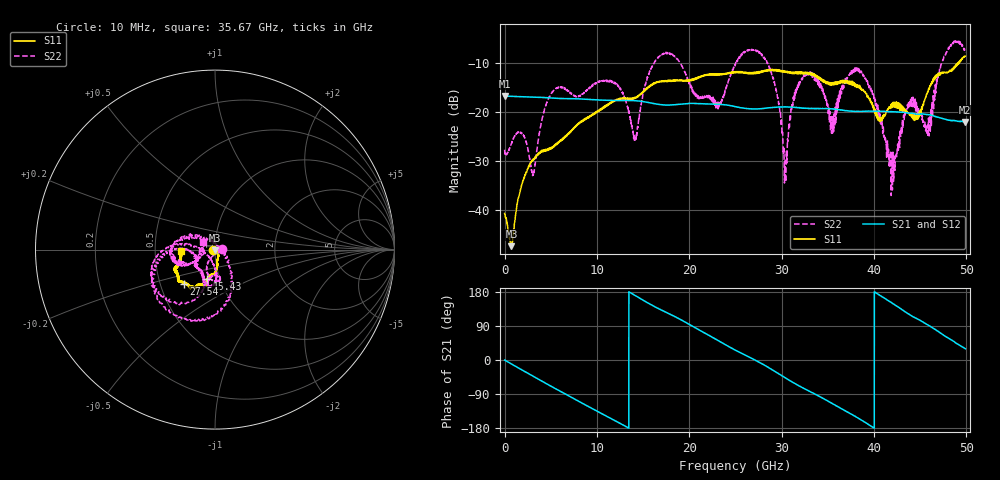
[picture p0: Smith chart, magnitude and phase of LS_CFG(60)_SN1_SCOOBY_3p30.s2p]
!Keysight Technologies,N5245B,MY58422026,A.13.80.08
!Date: Thursday, March 19, 2020 23:45:45
!Correction: S11(Full 2 Port(1,2))
!S21(Full 2 Port(1,2))
!S12(Full 2 Port(1,2))
!S22(Full 2 Port(1,2))
!S2P File: Measurements: S11, S21, S12, S22:
# Hz S DB R 50.0
!freq dBS11 angS11 dBS21 angS21 dBS12 angS12 dBS22 angS22
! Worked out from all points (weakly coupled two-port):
!   4991 points, 10 MHz to 49.91 GHz, reference 50 ohm
!   highest |S21| = -16.79 dB at 10 MHz (marker M1); lowest = -22.1 dB at 49.82 GHz (marker M2)
!   lowest |S11| = -47.4 dB at 750 MHz (marker M3), VSWR 1.01, Z = 49.8 - j0.367 ohm
!   |S11| at or under -10 dB: start of sweep to 49.13 GHz; 49.16379 GHz to 49.2268 GHz (63.01 MHz wide, 0.128 % of centre)
!   |S22| runs from -37.0 to -5.5 dB; largest |S21 - S12| = 0.0015
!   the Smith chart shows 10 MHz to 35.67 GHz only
!   S11 on the Smith chart (normalised r, x): 10 MHz: 0.98, -0.01; 15.43 GHz: 0.87, -0.30; 27.54 GHz: 0.66, -0.27; 35.67 GHz: 0.68, -0.01
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1e7  -40.71 -162.0  -16.79 -0.3  -16.77 -0.3  -27.72 0.9
7.5e8  -47.36 -120.7  -16.84 -10.5  -16.83 -10.5  -26.45 -29.2
2.8e9  -30.48 -55.0  -16.97 -38.6  -16.96 -38.6  -30.48 -29.9
5.15e9  -27.22 -66.6  -17.19 -70.8  -17.19 -70.7  -16.01 -101.9
8.33e9  -22.10 -81.1  -17.39 -113.0  -17.39 -112.9  -16.54 -95.8
1.208e10  -17.60 -89.0  -17.69 -161.5  -17.68 -161.4  -14.21 -91.3
1.412e10  -17.23 -97.6  -17.73 170.7  -17.73 170.8  -25.78 -138.5
1.543e10  -15.37 -104.3  -18.05 151.8  -18.05 151.9  -13.32 171.2
1.665e10  -13.95 -104.2  -18.46 135.9  -18.46 135.9  -8.93 -165.7
2.312e10  -12.50 -118.4  -18.44 51.7  -18.44 51.9  -19.39 -155.5
2.496e10  -12.00 -123.7  -18.91 26.5  -18.90 26.7  -10.55 -171.5
2.754e10  -11.83 -132.3  -19.38 -5.4  -19.38 -5.2  -7.82 -103.8
2.931e10  -11.51 -140.8  -19.07 -30.6  -19.07 -30.4  -14.71 -60.8
3.039e10  -11.81 -144.1  -19.01 -46.9  -19.01 -46.7  -31.25 44.2
3.148e10  -11.96 -150.0  -19.08 -62.6  -19.08 -62.3  -15.91 147.5
3.328e10  -12.31 -156.6  -19.31 -85.9  -19.32 -85.5  -12.25 -166.8
3.567e10  -14.38 -177.5  -19.43 -117.1  -19.37 -116.7  -22.23 147.2
3.839e10  -15.07 174.3  -19.93 -154.6  -19.87 -154.9  -11.33 -162.4
4.16e10  -19.12 106.2  -19.95 156.1  -19.97 156.0  -28.20 83.5
4.675e10  -12.50 7.4  -21.01 78.9  -21.03 79.1  -13.97 -136.6
4.982e10  -8.74 -15.1  -22.07 30.8  -22.08 30.9  -7.25 -13.3
4.991e10  -8.67 -14.2  -22.05 29.8  -22.08 29.8  -7.86 -13.6
